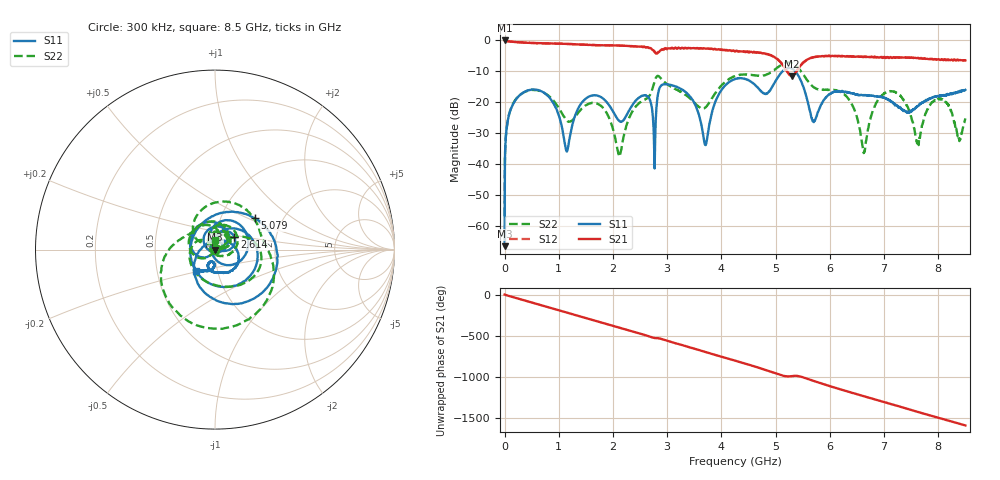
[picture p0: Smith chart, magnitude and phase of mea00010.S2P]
!Agilent Technologies,E5071B,MY42402595,A.08.01
!Date: Tue Jan 02 10:03:35 2001
!Data & Calibration Information:
!Freq	S11:SOLT2(ON)	S21:SOLT2(ON)	S12:SOLT2(ON)	S22:SOLT2(ON)
# Hz S dB R 50
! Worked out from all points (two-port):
!   1601 points, 300 kHz to 8.5 GHz, reference 50 ohm
!   highest |S21| = 0.01 dB at 300 kHz (marker M1); lowest = -11.5 dB at 5.297 GHz (marker M2)
!   |S21| within 3 dB of the highest: start of sweep to 2.726 GHz; 2.901 GHz to 3.975 GHz (1.074 GHz wide, 31.3 % of centre)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
!   lowest |S11| = -66.5 dB at 300 kHz (marker M3), VSWR 1.00, Z = 50 - j0.0365 ohm
!   |S11| at or under -10 dB: start of sweep to 5.126 GHz; 5.365 GHz to end of sweep
!   |S22| runs from -56.8 to -7.1 dB; largest |S21 - S12| = 0.026
!   S11 on the Smith chart (normalised r, x): 300 kHz: 1.00, -0.00; 2.614 GHz: 1.23, +0.17; 5.079 GHz: 1.45, +0.55; 8.5 GHz: 0.79, -0.19
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300000  -66.46 -50.2  0.01 0.1  -0.02 -0.1  -56.76 -131.8
5.873544e7  -25.94 -133.5  -0.23 -12.6  -0.23 -12.6  -25.89 -131.3
2.340418e8  -18.50 -171.7  -0.56 -46.3  -0.54 -46.3  -18.44 -164.3
8.874562e8  -19.89 41.2  -0.98 -168.7  -0.98 -168.7  -19.18 83.0
1.14776e9  -35.92 -94.2  -1.10 142.3  -1.09 142.3  -25.88 78.1
1.418687e9  -20.20 128.4  -1.32 91.4  -1.32 91.5  -22.11 95.7
1.955231e9  -21.62 35.1  -1.57 -8.6  -1.55 -8.7  -26.20 8.9
2.119913e9  -26.08 47.3  -1.64 -40.2  -1.65 -40.1  -36.98 55.7
2.613958e9  -17.83 32.9  -2.18 -135.3  -2.25 -135.6  -18.84 36.6
2.837075e9  -16.66 85.2  -3.82 -169.4  -3.71 -168.4  -11.48 -28.6
3.416117e9  -18.04 -42.8  -2.47 80.1  -2.47 80.2  -18.61 159.6
3.708294e9  -33.81 -180.0  -2.65 23.4  -2.61 23.4  -21.59 150.3
4.25015e9  -12.45 -5.4  -3.49 -80.5  -3.42 -80.7  -11.51 86.5
4.701697e9  -15.87 -129.3  -4.01 -169.5  -3.90 -169.3  -11.42 19.1
5.078871e9  -10.93 38.0  -6.81 108.1  -6.78 108.0  -8.18 -37.4
5.296676e9  -9.04 -46.6  -11.51 92.6  -11.49 91.9  -7.30 -104.9
5.668537e9  -25.20 141.9  -5.53 41.0  -5.61 41.1  -14.60 158.1
6.31664e9  -16.76 -59.4  -5.04 -91.7  -5.17 -91.9  -18.29 54.5
6.630066e9  -17.66 -79.9  -5.28 -152.0  -5.20 -151.1  -35.97 74.6
7.086925e9  -19.17 -110.0  -5.68 121.3  -5.44 121.0  -16.52 62.1
7.71909e9  -20.09 -95.0  -5.85 0.4  -5.86 -0.0  -26.49 139.9
8.5e9  -15.95 -132.0  -6.44 -145.5  -6.42 -146.4  -25.18 91.0
